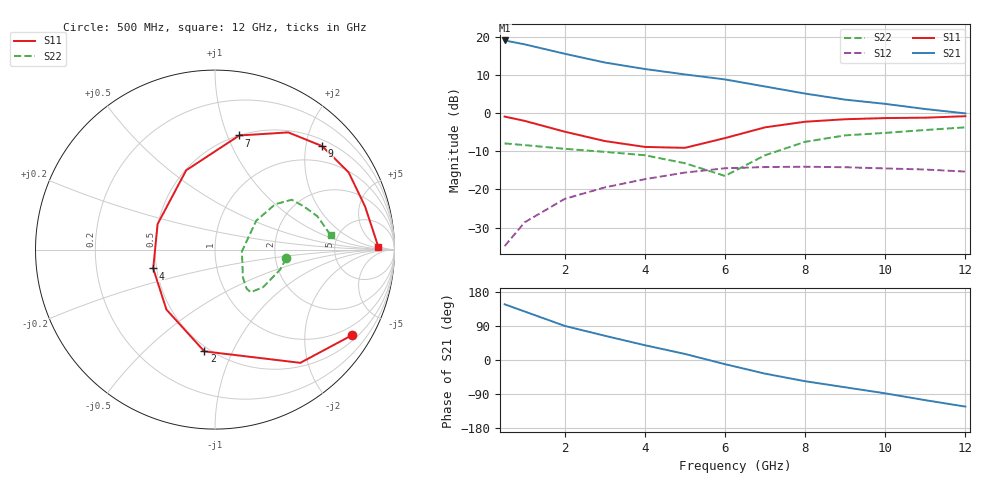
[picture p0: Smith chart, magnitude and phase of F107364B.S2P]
!ATF-10736
!S-PARAMETERS at Vds=4V  Id=70mA.  LAST UPDATED 07-22-92
# ghz s ma r 50
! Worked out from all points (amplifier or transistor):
!   13 points, 500 MHz to 12 GHz, reference 50 ohm
!   highest |S21| = 19.0 dB at 500 MHz (marker M1)
!   |S21| within 3 dB of that: start of sweep to 1.802 GHz
!   unconditionally stable (mu >= 1): 3.72 GHz to 7.17 GHz
!   at 2 GHz: K = 0.86, MSG = 19.0 dB, |S12| = -22.5 dB
!   at 6 GHz: K = 1.03, MAG = 10.6 dB, |S12| = -14.5 dB
!   at 12 GHz: K = 0.82, MSG = 7.6 dB, |S12| = -15.3 dB
!   S11 on the Smith chart (normalised r, x): 500 MHz: 0.67, -3.36; 2 GHz: 0.47, -0.79; 4 GHz: 0.48, -0.12; 7 GHz: 0.50, +1.10; 9 GHz: 0.63, +2.33; 12 GHz: 21, +4
0.5  0.9 -32.0  8.95 147.0  0.018 77.0  0.4 -7.0
1  0.79 -53.0  7.96 128.0  0.037 70.0  0.38 -17.0
2  0.57 -96.0  5.99 90.0  0.075 56.0  0.34 -38.0
3  0.43 -129.0  4.6 64.0  0.106 43.0  0.31 -50.0
4  0.36 -163.0  3.78 39.0  0.136 31.0  0.28 -51.0
5  0.35 156.0  3.21 16.0  0.166 14.0  0.22 -45.0
6  0.47 110.0  2.76 -11.0  0.189 -5.0  0.15 -4.0
7  0.65 78.0  2.23 -36.0  0.196 -23.0  0.28 35.0
8  0.77 58.0  1.8 -56.0  0.198 -38.0  0.42 37.0
9  0.83 44.0  1.5 -72.0  0.195 -48.0  0.51 33.0
10  0.86 30.0  1.32 -88.0  0.188 -64.0  0.55 26.0
11  0.87 16.0  1.13 -106.0  0.182 -77.0  0.6 18.0
12  0.91 1.0  0.99 -123.0  0.171 -91.0  0.65 7.0
